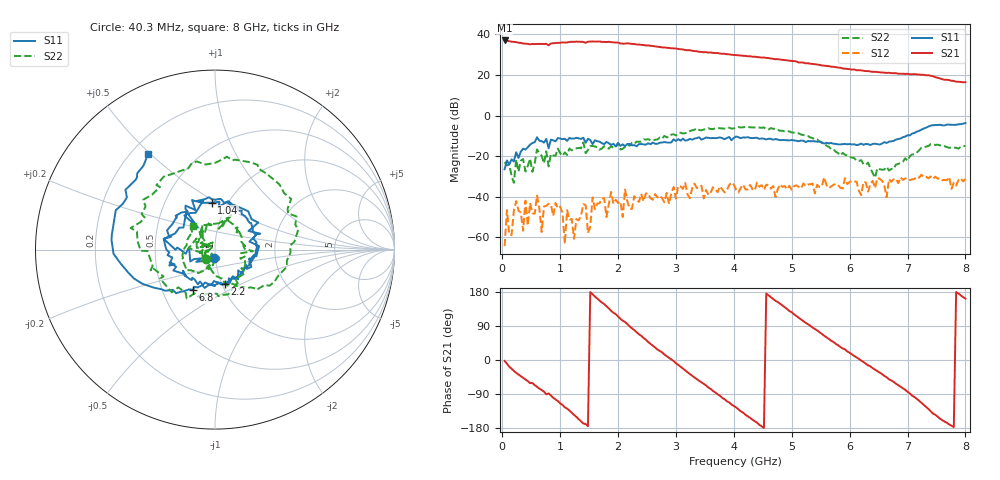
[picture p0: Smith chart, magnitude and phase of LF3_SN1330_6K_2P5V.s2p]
! VC=2.5V I=19.9mA
# HZ S DB R 50.00
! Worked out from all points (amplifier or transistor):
!   200 points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, 40.3 MHz to 8 GHz, reference 50 ohm
!   highest |S21| = 37.0 dB at 40.3 MHz (marker M1)
!   |S21| within 3 dB of that: start of sweep to 2.659 GHz
!   unconditionally stable (mu >= 1): start of sweep to 2.951 GHz; 3.386 GHz to 3.629 GHz; 4.415 GHz to end of sweep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
!   at 1.36 GHz: K = 2.16, MAG = 36.6 dB, |S12| = -49.2 dB
!   at 4.04 GHz: K = 1.04, MAG = 32.0 dB, |S12| = -36.6 dB
!   at 8 GHz: K = 1.70, MAG = 18.9 dB, |S12| = -31.2 dB
!   S11 on the Smith chart (normalised r, x): 40.3 MHz: 0.98, -0.09; 1.04 GHz: 0.84, +0.47; 2.2 GHz: 1.03, -0.41; 6.8 GHz: 0.72, -0.34; 8 GHz: 0.26, +0.49
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4.02985e7  -26.46 -98.0  36.96 -2.4  -64.33 8.1  -22.95 -135.0
2.002925e8  -22.62 -124.6  36.29 -28.6  -46.87 83.0  -33.13 108.6
4.00285e8  -16.76 174.7  35.38 -51.5  -41.94 163.0  -27.57 142.4
8.0027e8  -16.12 127.9  34.58 -88.0  -43.46 155.5  -25.06 148.9
1.040261e9  -11.64 93.9  36.02 -118.3  -48.05 -58.3  -19.89 133.1
1.400248e9  -10.92 32.0  36.25 -167.8  -43.60 -8.4  -13.26 63.8
1.680237e9  -12.84 -8.1  36.46 156.8  -43.20 17.8  -16.86 36.5
1.920228e9  -13.92 -41.3  36.00 124.7  -43.42 -4.2  -15.95 8.6
2.200218e9  -13.98 -74.4  35.42 88.8  -45.89 -12.1  -14.92 -35.3
2.520206e9  -13.65 -109.1  34.51 47.4  -38.30 -53.4  -11.69 -85.9
2.720198e9  -13.40 -127.5  33.75 24.0  -39.39 -71.5  -10.87 -103.7
3.000188e9  -12.52 -156.2  33.03 -8.7  -40.95 -100.7  -9.81 -152.5
3.360174e9  -11.13 175.6  31.66 -50.5  -35.71 -72.1  -6.29 165.6
3.72016e9  -10.99 139.0  30.76 -90.5  -37.77 -160.6  -6.07 125.0
4.040148e9  -10.32 114.8  29.78 -125.2  -36.60 -150.6  -5.95 85.3
4.52013e9  -11.42 73.4  28.56 -179.4  -36.56 150.2  -5.86 33.6
4.960114e9  -12.25 37.3  27.00 129.2  -34.60 104.9  -7.84 -14.9
5.360099e9  -12.64 3.0  25.41 85.6  -33.52 76.6  -11.07 -50.4
5.960076e9  -14.17 -44.3  22.92 22.4  -33.73 27.0  -19.79 -114.4
6.68005e9  -12.86 -113.7  21.07 -50.9  -31.30 -31.3  -27.09 -63.9
6.800045e9  -11.88 -118.4  20.84 -62.5  -31.05 -45.2  -24.17 -68.2
8e9  -3.73 125.2  16.40 161.9  -31.25 -134.4  -14.89 134.0
